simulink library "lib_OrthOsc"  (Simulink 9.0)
settings: Solver=ode45  StartTime=0.0  StopTime=10.0  RelTol=1e-3  EnableMultiTasking=on
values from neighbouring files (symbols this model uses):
  Tinit = 0.100    (= 0.1)    [TestOrthOscObjO_init.m]    (also in TestWaveMng_init.m)
  Tstep = 0.0005    [TestOrthOscObjO_init.m]    (also in TestWaveMng_init.m = 5e-05)
undefined symbols (not defined in the file or in its folder): Fmax, Fmin, Fnom, K, maxError, minMagn, src2genBus, Tg, TP, Tstep_
libraries: lib_T1Blocks_FB x5, lib_Conv x5, lib_Ortholator x2, lib_AngleVectorBlocks x2, lib_Inspc x1

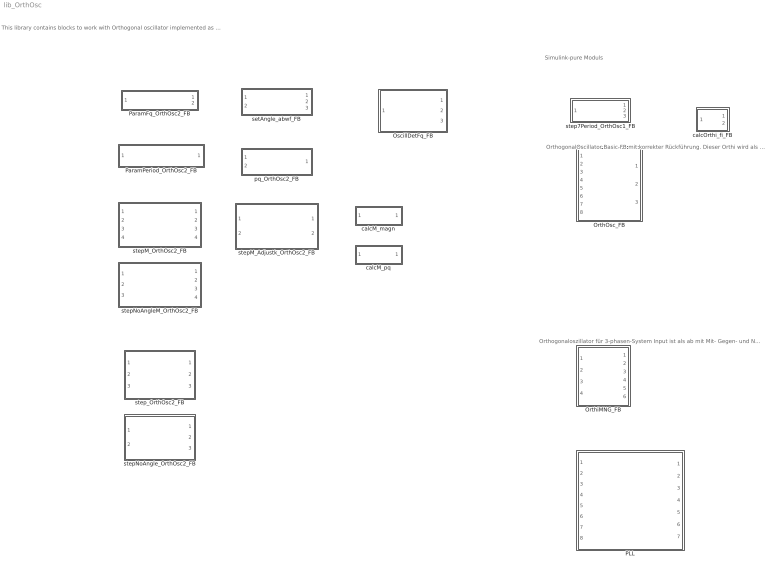
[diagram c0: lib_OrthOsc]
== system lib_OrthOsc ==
  note: Simulink-pure Moduls
  note: This library contains blocks to work with Orthogonal oscillator implemented as S-Function
  note: Orthogonaloszillator für 3-phasen-System Input ist als ab mit Mit- Gegen- und Nullsystem gegeben. Orthi separiert Gleichanteil (yG), Mitsystem(yM) und Gegensystem (yN) date=2016-03-04
  note: OrthogonalOscillator Basic-FB mit korrekter Rückführung. Dieser Orthi wird als Basis in den anderen FB verwendet.
  OrthOsc_FB : Subsystem
  OrthiMNG_FB : Subsystem
  OscillDetFq_FB : Subsystem
  PLL : Subsystem
  ParamFq_OrthOsc2_FB : Subsystem
  ParamPeriod_OrthOsc2_FB : Subsystem
  calcM_magn : Subsystem  TreatAsAtomicUnit=on
  calcM_pq : Subsystem  TreatAsAtomicUnit=on
  calcOrthi_fi_FB : Subsystem
  pq_OrthOsc2_FB : Subsystem
  setAngle_abwf_FB : Subsystem
  step7Period_OrthOsc1_FB : Subsystem
  stepM_Adjustk_OrthOsc2_FB : Subsystem  TreatAsAtomicUnit=on
  stepM_OrthOsc2_FB : Subsystem  TreatAsAtomicUnit=on
  stepNoAngleM_OrthOsc2_FB : Subsystem  TreatAsAtomicUnit=on
  stepNoAngle_OrthOsc2_FB : Subsystem
  step_OrthOsc2_FB : Subsystem  LoadFcn=src2genBus.lib_OrthOsc_genBus();

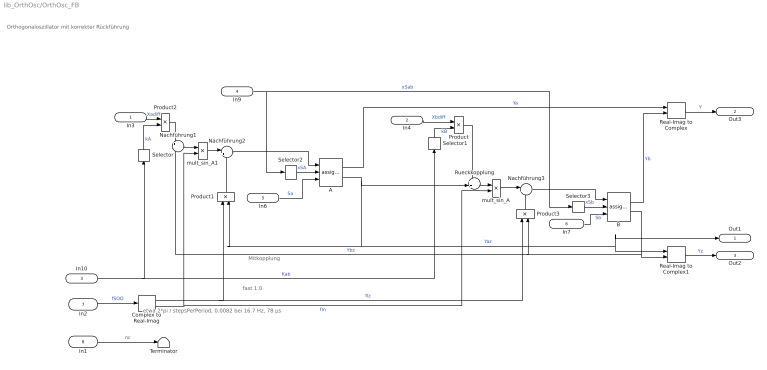
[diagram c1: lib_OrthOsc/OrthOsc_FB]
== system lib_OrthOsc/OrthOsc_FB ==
  note: Orthogonaloszillator mit korrekter Rückführung
  note: fast 1.0
  note: etwa 2*pi / stepsPerPeriod, 0.0082 bei 16.7 Hz, 78 µs
  note: Mitkopplung
  In3 : Inport
  In4 : Inport  Port=2
  In10 : Inport  Port=3  OutDataTypeStr=single  PortDimensions=2
  In9 : Inport  Port=4
  In6 : Inport  Port=5  OutDataTypeStr=boolean
  In7 : Inport  Port=6  OutDataTypeStr=boolean
  In2 : Inport  Port=7  OutDataTypeStr=single
  In1 : Inport  Port=8  OutDataTypeStr=boolean
  A : lib_T1Blocks_FB/assignS_OpC
  B : lib_T1Blocks_FB/assignS_OpC
  Complex to Real-Imag : ComplexToRealImag
  Nachführung1 : Sum  Inputs=+|-
  Nachführung2 : Sum  Inputs=|++
  Nachführung3 : Sum  Inputs=|++
  Product{,1..3} (4 alike) : Product
  Real-Imag to Complex : RealImagToComplex
  Real-Imag to Complex1 : RealImagToComplex
  Rueckkopplung : Sum  Inputs=++|
  Selector : Selector  InputPortWidth=2  IndexOptions=Index vector (dialog)  Indices=[1]  OutputSizes=1
  Selector1 : Selector  InputPortWidth=2  IndexOptions=Index vector (dialog)  Indices=[2]  OutputSizes=1
  Selector2 : Selector  InputPortWidth=2  IndexOptions=Index vector (dialog)  Indices=[1]  OutputSizes=1
  Selector3 : Selector  InputPortWidth=2  IndexOptions=Index vector (dialog)  Indices=[2]  OutputSizes=1
  Terminator : Terminator
  mult_sin_A : Product
  mult_sin_A1 : Product
  Out1 : Outport
  Out3 : Outport  Port=2
  Out2 : Outport  Port=3
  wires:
  In1/1 -> Terminator/1  "nc"
  In9/1 -> Selector2/1, Selector3/1  "xSab"
  In10/1 -> Selector1/1, Selector/1  "Kab"
  Real-Imag to Complex1/1 -> Out2/1  "Yz"
  B/1 -> Real-Imag to Complex/2  "Yb"
  Complex to Real-Imag/1 -> Product3/1, Product1/1  "fIz"
  Product3/1 -> Nachführung3/2
  Nachführung3/1 -> B/1
  Product1/1 -> Nachführung2/2
  Nachführung2/1 -> A/1
  Selector2/1 -> A/2  "xSA"
  Selector3/1 -> B/2  "xSb"
  In7/1 -> B/3  "Sb"
  Selector1/1 -> Product/2  "kB"
  In4/1 -> Product/1  "Xbdiff"
  In6/1 -> A/3  "Sa"
  Selector/1 -> Product2/2  "kA"
  B/2 -> Real-Imag to Complex1/2, Product3/2, Nachführung1/2  "Ybz"
  A/1 -> Real-Imag to Complex/1  "Ya"
  mult_sin_A/1 -> Nachführung3/1
  Rueckkopplung/1 -> mult_sin_A/1
  In2/1 -> Complex to Real-Imag/1  "fSOO"
  Product/1 -> Rueckkopplung/1
  In3/1 -> Product2/1  "Xadiff"
  Product2/1 -> Nachführung1/1
  A/2 -> Rueckkopplung/2, Real-Imag to Complex1/1, Out1/1, Product1/2  "Yaz"
  Nachführung1/1 -> mult_sin_A1/1
  mult_sin_A1/1 -> Nachführung2/1
  Real-Imag to Complex/1 -> Out3/1  "Y"
  Complex to Real-Imag/2 -> mult_sin_A/2, mult_sin_A1/2  "fIn"

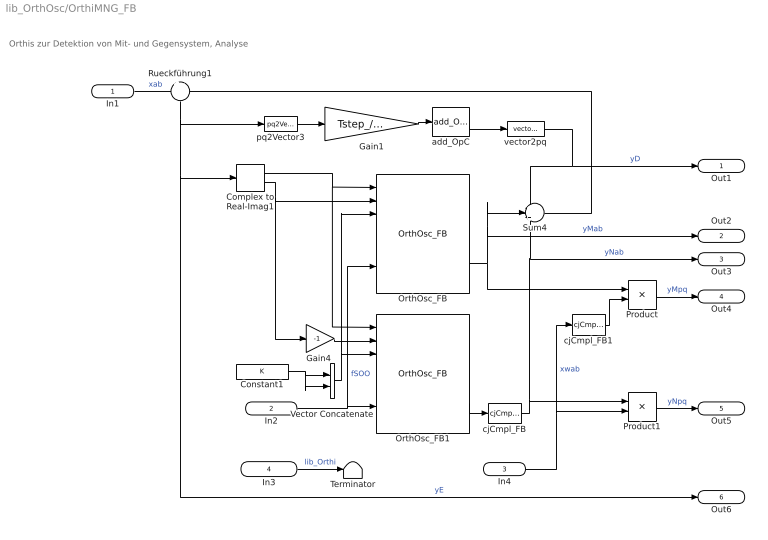
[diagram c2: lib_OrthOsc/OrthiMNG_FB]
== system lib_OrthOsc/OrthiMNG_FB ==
  note: Orthis zur Detektion von Mit- und Gegensystem, Analyse
  In1 : Inport  OutDataTypeStr=single
  In2 : Inport  Port=2  OutDataTypeStr=single
  In4 : Inport  Port=3  OutDataTypeStr=single
  In3 : Inport  Port=4  OutDataTypeStr=boolean
  Complex to Real-Imag1 : ComplexToRealImag
  Constant1 : Constant  Value=K  OutDataTypeStr=single
  Gain1 : Gain  Gain=Tstep_/Tg
  Gain4 : Gain  Gain=-1
  OrthOsc_FB : lib_Ortholator/OrthOsc_FB
  OrthOsc_FB1 : lib_Ortholator/OrthOsc_FB
  Product : Product
  Product1 : Product
  Rueckführung1 : Sum  Inputs=+-
  Sum4 : Sum  Inputs=+++
  Terminator : Terminator
  Vector Concatenate : Concatenate
  add_OpC : lib_T1Blocks_FB/add_OpC  y0=0
  cjCmpl_FB : lib_Conv/cjCmpl_FB
  cjCmpl_FB1 : lib_Conv/cjCmpl_FB
  pq2Vector3 : lib_Conv/pq2Vector  SystemSampleTime=-1
  vector2pq : lib_Conv/vector2pq  SystemSampleTime=-1
  Out1 : Outport  OutDataTypeStr=single
  Out2 : Outport  Port=2  OutDataTypeStr=single
  Out3 : Outport  Port=3  OutDataTypeStr=single
  Out4 : Outport  Port=4  OutDataTypeStr=single
  Out5 : Outport  Port=5  OutDataTypeStr=single
  Out6 : Outport  Port=6  OutDataTypeStr=single
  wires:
  Product1/1 -> Out5/1  "yNpq"
  Product/1 -> Out4/1  "yMpq"
  In4/1 -> Product1/2, cjCmpl_FB1/1  "xwab"
  cjCmpl_FB1/1 -> Product/2
  OrthOsc_FB1/3 -> cjCmpl_FB/1
  cjCmpl_FB/1 -> Product1/1, Sum4/3, Out3/1  "yNab"
  Sum4/1 -> Rueckführung1/2
  OrthOsc_FB/3 -> Product/1, Out2/1, Sum4/2  "yMab"
  In2/1 -> OrthOsc_FB/7, OrthOsc_FB1/7  "fSOO"
  Gain1/1 -> add_OpC/1
  In1/1 -> Rueckführung1/1  "xab"
  Rueckführung1/1 -> Out6/1, Complex to Real-Imag1/1, pq2Vector3/1  "yE"
  Vector Concatenate/1 -> OrthOsc_FB1/3, OrthOsc_FB/3
  vector2pq/1 -> Out1/1, Sum4/1  "yD"
  Complex to Real-Imag1/1 -> OrthOsc_FB1/1, OrthOsc_FB/1
  pq2Vector3/1 -> Gain1/1
  add_OpC/2 -> vector2pq/1
  Complex to Real-Imag1/2 -> Gain4/1, OrthOsc_FB/2
  Gain4/1 -> OrthOsc_FB1/2
  Constant1/1 -> Vector Concatenate/2, Vector Concatenate/1
  In3/1 -> Terminator/1  "lib_Orthi"

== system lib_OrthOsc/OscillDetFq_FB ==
  In1 : Inport  OutDataTypeStr=single  PortDimensions=1
  SFunc : S-Function  LoadFcn=src2genBus.lib_OrthOsc_genBus();  FunctionName=step_OscillDetFq_FB_SfH  Parameters=ident Tstep dxstart dxmin amplMin stepNom stepMax  SFunctionDeploymentMode=off  EnableBusSupport=off
  Out4 : Outport  OutDataTypeStr=uint32  SampleTime=Tinit
  Out1 : Outport  Port=2  OutDataTypeStr=uint32
  Out3 : Outport  Port=3  OutDataTypeStr=single
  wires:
  SFunc/2 -> Out1/1  "thiz"
  In1/1 -> SFunc/1  "X"
  SFunc/3 -> Out3/1  "nSteps"
  SFunc/1 -> Out4/1  "OscillDetFq_FB"

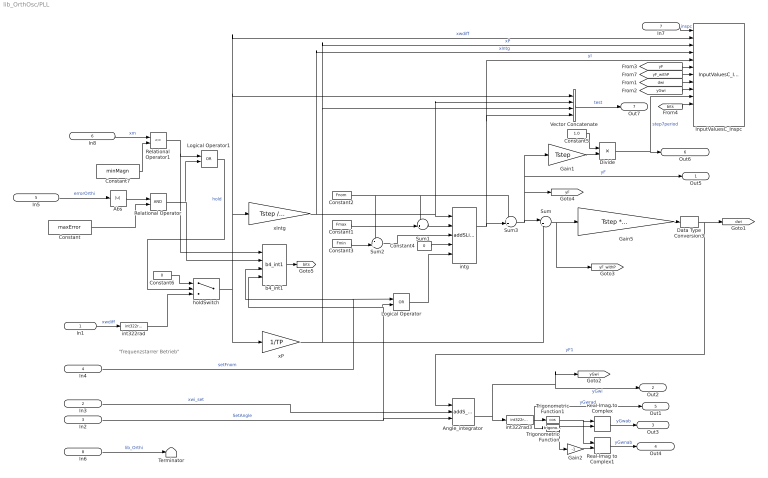
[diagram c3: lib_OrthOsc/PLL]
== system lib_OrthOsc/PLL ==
  note: "frequenzstarrer Betrieb"
  In1 : Inport
  In3 : Inport  Port=2  OutDataTypeStr=int32
  In2 : Inport  Port=3  OutDataTypeStr=boolean
  In4 : Inport  Port=4  OutDataTypeStr=boolean
  In5 : Inport  Port=5  OutDataTypeStr=single  PortDimensions=1
  In8 : Inport  Port=6  OutDataTypeStr=single  PortDimensions=1
  In7 : Inport  Port=7  OutDataTypeStr=P_FBaccess_Inspc  PortDimensions=1  SampleTime=Tstep
  In6 : Inport  Port=8  OutDataTypeStr=boolean
  Abs : Abs
  Angle_integrator : lib_T1Blocks_FB/addS_OpC
  Constant : Constant  Value=maxError
  Constant1 : Constant  Value=Fmax  OutDataTypeStr=single
  Constant2 : Constant  Value=Fnom  OutDataTypeStr=single
  Constant3 : Constant  Value=Fmin  OutDataTypeStr=single
  Constant4 : Constant  Value=0  OutDataTypeStr=single
  Constant5 : Constant  Value=1.0  OutDataTypeStr=single
  Constant6 : Constant  Value=0  OutDataTypeStr=single
  Constant7 : Constant  Value=minMagn
  Data Type Conversion3 : DataTypeConversion  OutDataTypeStr=int32
  Divide : Product  Inputs=*/
  Gain1 : Gain  Gain=Tstep
  Gain2 : Gain  Gain=-1
  Gain5 : Gain  Gain=Tstep * 65536 * 65536
  InputValuesC_Inspc : lib_Inspc/InputValuesC_Inspc  nameRefl=nameInspc  n1='wxdiff_rad'  n2='xP'  n3='xIntg'  n4='yIntg'  n5='yF'  n6='yF_withP'  n7='dwi'  n8='yGwi'  n9='step7period'  n10='hold_setG_setF_err_magn'  n11=''  n12=''
  Logical Operator : Logic  Operator=OR  IconShape=distinctive  AllPortsSameDT=off  OutDataTypeStr=boolean
  Logical Operator1 : Logic  Operator=OR  AllPortsSameDT=off  OutDataTypeStr=boolean
  Real-Imag to Complex : RealImagToComplex
  Real-Imag to Complex1 : RealImagToComplex
  Relational Operator : RelationalOperator  OutDataTypeStr=boolean
  Relational Operator1 : RelationalOperator  Operator=<=  OutDataTypeStr=boolean
  Sum : Sum  Inputs=|++
  Sum1 : Sum  Inputs=-+|
  Sum2 : Sum  Inputs=-+|
  Sum3 : Sum  Inputs=++|
  Terminator : Terminator
  Trigonometric Function : Trigonometry
  Trigonometric Function1 : Trigonometry  Operator=cos
  Vector Concatenate : Concatenate  NumInputs=4
  b4_int1 : lib_Conv/b4_int1  b0bit=0  b1bit=1  b2bit=2  b3bit=3
  holdSwitch : Switch
  int322rad : lib_AngleVectorBlocks/int322rad
  int322rad3 : lib_AngleVectorBlocks/int322rad
  intg : lib_T1Blocks_FB/addSLim_OpC
  xIntg : Gain  Gain=Tstep / Tintg
  xP : Gain  Gain=1/TP
  Out5 : Outport  OutDataTypeStr=single  PortDimensions=1
  Out2 : Outport  Port=2  OutDataTypeStr=int32  PortDimensions=1
  Out3 : Outport  Port=3  OutDataTypeStr=single  PortDimensions=1
  Out4 : Outport  Port=4  OutDataTypeStr=single  PortDimensions=1
  Out1 : Outport  Port=5  OutDataTypeStr=single  PortDimensions=1
  Out6 : Outport  Port=6  OutDataTypeStr=single  PortDimensions=1
  Out7 : Outport  Port=7  OutDataTypeStr=single  PortDimensions=4
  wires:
  [bits] -> InputValuesC_Inspc/11
  b4_int1/1 -> [bits]
  [yF] -> InputValuesC_Inspc/6
  In8/1 -> Relational Operator1/1  "xm"
  Relational Operator/1 -> b4_int1/2, Logical Operator1/2
  Relational Operator1/1 -> b4_int1/1, Logical Operator1/1
  Constant7/1 -> Relational Operator1/2
  Constant/1 -> Relational Operator/2
  Abs/1 -> Relational Operator/1
  In5/1 -> Abs/1  "errorOrthi"
  [yGwi] -> InputValuesC_Inspc/9
  [dwi] -> InputValuesC_Inspc/8
  [yF_withP] -> InputValuesC_Inspc/7
  In7/1 -> InputValuesC_Inspc/1  "inspc"
  int322rad/1 -> holdSwitch/3
  Constant6/1 -> holdSwitch/1
  Vector Concatenate/1 -> Out7/1  "test"
  In6/1 -> Terminator/1  "lib_Orthi"
  holdSwitch/1 -> Vector Concatenate/1, InputValuesC_Inspc/2, xIntg/1, xP/1  "xwdiff"
  Logical Operator1/1 -> holdSwitch/2  "hold"
  In4/1 -> Logical Operator/1, b4_int1/3  "setFnom"
  Logical Operator/1 -> intg/5
  Divide/1 -> Out6/1, InputValuesC_Inspc/10  "step7period"
  Constant5/1 -> Divide/1
  Gain1/1 -> Divide/2
  In3/1 -> Angle_integrator/2  "xwi_set"
  In2/1 -> b4_int1/4, Logical Operator/2, Angle_integrator/3  "SetAngle"
  xIntg/1 -> Vector Concatenate/2, intg/1, InputValuesC_Inspc/4  "xIntg"
  xP/1 -> Sum/2, Vector Concatenate/3, InputValuesC_Inspc/3  "xP"
  In1/1 -> int322rad/1  "xwdiff"
  Constant4/1 -> intg/4
  Constant3/1 -> Sum2/2
  Sum2/1 -> intg/3
  Sum1/1 -> intg/2
  Constant2/1 -> Sum3/1, Sum1/1, Sum2/1
  Sum/1 -> Gain5/1, [yF_withP]
  Data Type Conversion3/1 -> Angle_integrator/1, [dwi]  "yF1"
  Constant1/1 -> Sum1/2
  intg/1 -> Sum3/2, Vector Concatenate/4, InputValuesC_Inspc/5  "yI"
  Gain5/1 -> Data Type Conversion3/1
  Real-Imag to Complex1/1 -> Out4/1  "yGwnab"
  Real-Imag to Complex/1 -> Out3/1  "yGwab"
  Gain2/1 -> Real-Imag to Complex1/2
  Trigonometric Function/1 -> Real-Imag to Complex/2, Gain2/1
  Trigonometric Function1/1 -> Real-Imag to Complex/1, Real-Imag to Complex1/1
  int322rad3/1 -> Trigonometric Function1/1, Trigonometric Function/1, Out1/1  "yGwrad"
  Angle_integrator/2 -> int322rad3/1, Out2/1, [yGwi]  "yGwi"
  Sum3/1 -> Out5/1, Gain1/1, [yF], Sum/1  "yF"

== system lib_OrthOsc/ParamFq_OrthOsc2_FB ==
  In1 : Inport  OutDataTypeStr=single
  param1_myOrthOsc : S-Function  FunctionName=setFq_Param_OrthOsc2_FB_SfH  Parameters=identObj Tstep TstepOrth m_nom  SFunctionDeploymentMode=off  EnableBusSupport=off
  Out2 : Outport  OutDataTypeStr=uint32  SampleTime=Tinit
  Out1 : Outport  Port=2  OutDataTypeStr=uint32  SampleTime=Tstep
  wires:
  In1/1 -> param1_myOrthOsc/1  "fq"
  param1_myOrthOsc/1 -> Out2/1  "Param_OrthOsc2_FB"
  param1_myOrthOsc/2 -> Out1/1  "thiz"

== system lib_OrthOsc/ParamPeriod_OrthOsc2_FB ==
  In1 : Inport  OutDataTypeStr=single
  sfn : S-Function  FunctionName=setPeriod_Param_OrthOsc2_FB_SfH  Parameters=identObj Tstep TstepOrth m_nom  SFunctionDeploymentMode=off  EnableBusSupport=off
  Out2 : Outport  OutDataTypeStr=uint32
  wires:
  sfn/1 -> Out2/1  "Param_OrthOsc2_FB"
  In1/1 -> sfn/1  "nPeriod"

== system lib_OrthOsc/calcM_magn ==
  In1 : Inport  OutDataTypeStr=uint32  Partition=on  PartitionDimension=1  PartitionWidth=1  PartitionOffset=0
  For Each : ForEach  DisableCoverage=on  IndexMode=One-based
  calcMagn_Orthi2_FB : S-Function  FunctionName=calcMagn_OrthOsc2_FB_SfH  SFunctionDeploymentMode=off  EnableBusSupport=off
  Out3 : Outport  OutDataTypeStr=single  ConcatenationDimension=1
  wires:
  In1/1 -> calcMagn_Orthi2_FB/1  "thiz"
  calcMagn_Orthi2_FB/1 -> Out3/1  "ym"

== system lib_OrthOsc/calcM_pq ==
  In1 : Inport  OutDataTypeStr=uint32  Partition=on  PartitionDimension=1  PartitionWidth=1  PartitionOffset=0
  For Each : ForEach  DisableCoverage=on  IndexMode=One-based
  step_Orthi2_FB : S-Function  FunctionName=calcpq_OrthOsc2_FB_SfH  SFunctionDeploymentMode=off  EnableBusSupport=off
  Out3 : Outport  OutDataTypeStr=single  ConcatenationDimension=1
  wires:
  In1/1 -> step_Orthi2_FB/1  "thiz"
  step_Orthi2_FB/1 -> Out3/1  "ypq"

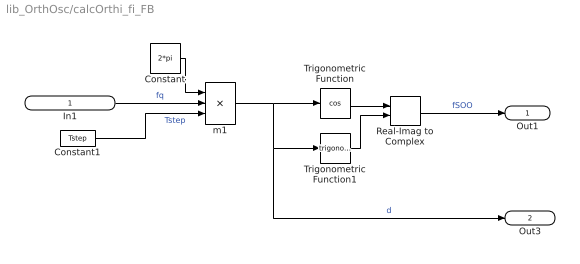
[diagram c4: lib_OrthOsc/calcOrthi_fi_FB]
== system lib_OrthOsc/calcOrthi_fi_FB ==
  In1 : Inport  OutDataTypeStr=single
  Constant : Constant  Value=2*pi  OutDataTypeStr=single
  Constant1 : Constant  Value=Tstep  OutDataTypeStr=single
  Real-Imag to Complex : RealImagToComplex
  Trigonometric Function : Trigonometry  Operator=cos
  Trigonometric Function1 : Trigonometry
  m1 : Product  Inputs=***
  Out1 : Outport
  Out3 : Outport  Port=2
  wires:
  Constant1/1 -> m1/3  "Tstep"
  Constant/1 -> m1/1
  m1/1 -> Trigonometric Function/1, Trigonometric Function1/1, Out3/1  "d"
  In1/1 -> m1/2  "fq"
  Real-Imag to Complex/1 -> Out1/1  "fSOO"
  Trigonometric Function1/1 -> Real-Imag to Complex/2
  Trigonometric Function/1 -> Real-Imag to Complex/1

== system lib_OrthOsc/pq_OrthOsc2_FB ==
  In3 : Inport  OutDataTypeStr=uint32
  In2 : Inport  Port=2  OutDataTypeStr=single
  calcpq_OrthOsc2_FB : S-Function  FunctionName=calcpq_OrthOsc2_FB_SfH  SFunctionDeploymentMode=off  EnableBusSupport=off
  thiz_Angle_abwmf_FB : Outport  OutDataTypeStr=single
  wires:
  In3/1 -> calcpq_OrthOsc2_FB/1  "thiz_OrthOs2_FB"
  In2/1 -> calcpq_OrthOsc2_FB/2  "step"
  calcpq_OrthOsc2_FB/1 -> thiz_Angle_abwmf_FB/1  "pq"

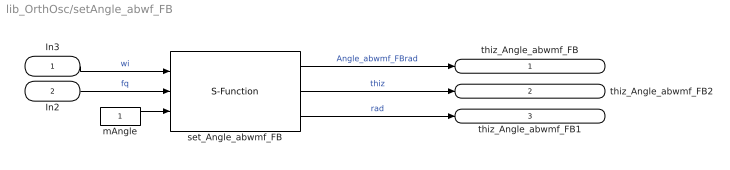
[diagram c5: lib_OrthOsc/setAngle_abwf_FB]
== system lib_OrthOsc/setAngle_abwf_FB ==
  In3 : Inport  OutDataTypeStr=int32
  In2 : Inport  Port=2  OutDataTypeStr=single
  mAngle : Constant  OutDataTypeStr=single
  set_Angle_abwmf_FB : S-Function  FunctionName=set_Angle_abwmf_FB_SfH  Parameters=identObj  SFunctionDeploymentMode=off  EnableBusSupport=off
  thiz_Angle_abwmf_FB : Outport  OutDataTypeStr=uint32  SampleTime=Tinit
  thiz_Angle_abwmf_FB2 : Outport  Port=2  OutDataTypeStr=uint32  SampleTime=Tstep
  thiz_Angle_abwmf_FB1 : Outport  Port=3  OutDataTypeStr=single
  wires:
  In3/1 -> set_Angle_abwmf_FB/1  "wi"
  In2/1 -> set_Angle_abwmf_FB/2  "fq"
  mAngle/1 -> set_Angle_abwmf_FB/3
  set_Angle_abwmf_FB/1 -> thiz_Angle_abwmf_FB/1  "Angle_abwmf_FBrad"
  set_Angle_abwmf_FB/3 -> thiz_Angle_abwmf_FB1/1  "rad"
  set_Angle_abwmf_FB/2 -> thiz_Angle_abwmf_FB2/1  "thiz"

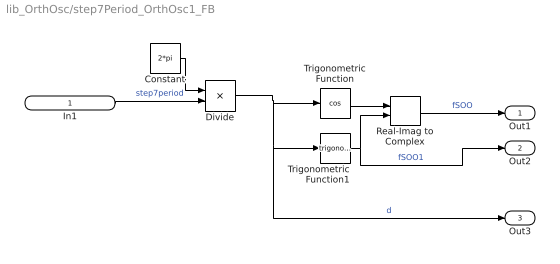
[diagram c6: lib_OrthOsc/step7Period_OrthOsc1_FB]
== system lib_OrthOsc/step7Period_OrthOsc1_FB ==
  In1 : Inport  OutDataTypeStr=single
  Constant : Constant  Value=2*pi  OutDataTypeStr=single
  Divide : Product  Inputs=*/
  Real-Imag to Complex : RealImagToComplex
  Trigonometric Function : Trigonometry  Operator=cos
  Trigonometric Function1 : Trigonometry
  Out1 : Outport
  Out2 : Outport  Port=2
  Out3 : Outport  Port=3
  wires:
  Trigonometric Function/1 -> Real-Imag to Complex/1
  Trigonometric Function1/1 -> Real-Imag to Complex/2, Out2/1  "fSOO1"
  Real-Imag to Complex/1 -> Out1/1  "fSOO"
  In1/1 -> Divide/2  "step7period"
  Divide/1 -> Out3/1, Trigonometric Function1/1, Trigonometric Function/1  "d"
  Constant/1 -> Divide/1

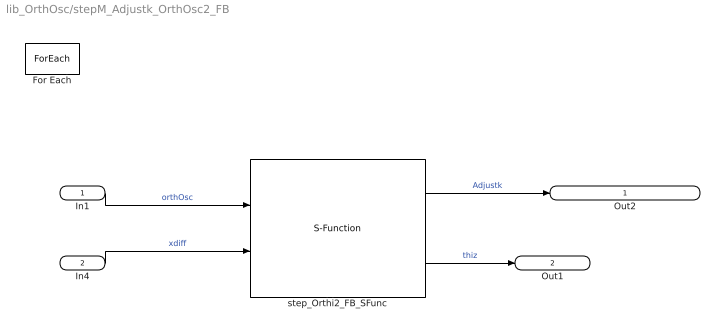
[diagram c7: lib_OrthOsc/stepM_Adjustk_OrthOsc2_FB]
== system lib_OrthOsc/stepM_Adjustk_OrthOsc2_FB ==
  In1 : Inport  OutDataTypeStr=uint32  PortDimensions=1  Partition=on  PartitionDimension=1  PartitionWidth=1  PartitionOffset=0
  In4 : Inport  Port=2  OutDataTypeStr=single  Partition=on  PartitionDimension=1  PartitionWidth=1  PartitionOffset=0
  For Each : ForEach  DisableCoverage=on  IndexMode=One-based
  step_Orthi2_FB_SFunc : S-Function  LoadFcn=src2genBus.lib_OrthOsc_genBus();  FunctionName=step_Adjustk_OrthOsc2_FB_SfH  Parameters=ident max_e kHi kNormal Tstep Tdecay  SFunctionDeploymentMode=off  EnableBusSupport=off
  Out2 : Outport  OutDataTypeStr=uint32  ConcatenationDimension=1
  Out1 : Outport  Port=2  OutDataTypeStr=uint32  ConcatenationDimension=1
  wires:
  In4/1 -> step_Orthi2_FB_SFunc/2  "xdiff"
  In1/1 -> step_Orthi2_FB_SFunc/1  "orthOsc"
  step_Orthi2_FB_SFunc/2 -> Out1/1  "thiz"
  step_Orthi2_FB_SFunc/1 -> Out2/1  "Adjustk"

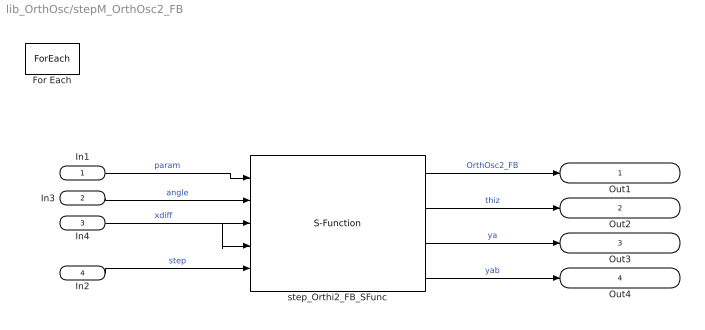
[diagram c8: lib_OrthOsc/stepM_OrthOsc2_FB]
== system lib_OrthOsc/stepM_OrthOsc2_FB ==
  In1 : Inport  OutDataTypeStr=uint32  PortDimensions=1
  In3 : Inport  Port=2  OutDataTypeStr=uint32
  In4 : Inport  Port=3  OutDataTypeStr=single  Partition=on  PartitionDimension=1  PartitionWidth=1  PartitionOffset=0
  In2 : Inport  Port=4  OutDataTypeStr=uint32  PortDimensions=1
  For Each : ForEach  DisableCoverage=on  IndexMode=One-based
  step_Orthi2_FB_SFunc : S-Function  LoadFcn=src2genBus.lib_OrthOsc_genBus();  FunctionName=step_OrthOsc2_FB_SfH  Parameters=ident kA kB  SFunctionDeploymentMode=off  EnableBusSupport=off
  Out1 : Outport  OutDataTypeStr=uint32  SampleTime=Tinit  ConcatenationDimension=1
  Out2 : Outport  Port=2  OutDataTypeStr=uint32  SampleTime=Tstep  ConcatenationDimension=1
  Out3 : Outport  Port=3  OutDataTypeStr=single  ConcatenationDimension=1
  Out4 : Outport  Port=4  OutDataTypeStr=single  ConcatenationDimension=1
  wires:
  In3/1 -> step_Orthi2_FB_SFunc/2  "angle"
  In1/1 -> step_Orthi2_FB_SFunc/1  "param"
  step_Orthi2_FB_SFunc/1 -> Out1/1  "OrthOsc2_FB"
  In4/1 -> step_Orthi2_FB_SFunc/4, step_Orthi2_FB_SFunc/3  "xdiff"
  step_Orthi2_FB_SFunc/3 -> Out3/1  "ya"
  step_Orthi2_FB_SFunc/4 -> Out4/1  "yab"
  step_Orthi2_FB_SFunc/2 -> Out2/1  "thiz"
  In2/1 -> step_Orthi2_FB_SFunc/5  "step"

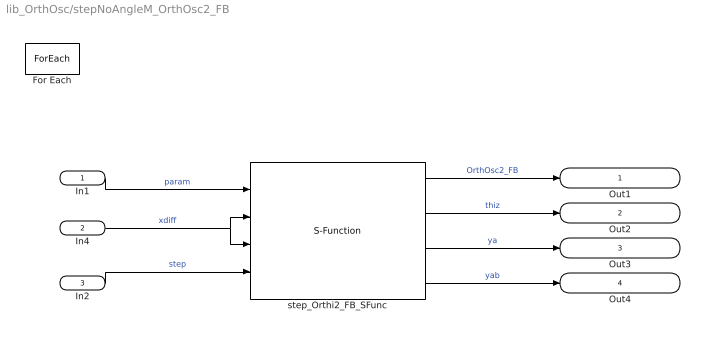
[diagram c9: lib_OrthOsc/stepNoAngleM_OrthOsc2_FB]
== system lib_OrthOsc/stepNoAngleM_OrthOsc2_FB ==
  In1 : Inport  OutDataTypeStr=uint32  PortDimensions=1
  In4 : Inport  Port=2  OutDataTypeStr=single  Partition=on  PartitionDimension=1  PartitionWidth=1  PartitionOffset=0
  In2 : Inport  Port=3  OutDataTypeStr=uint32  PortDimensions=1
  For Each : ForEach  DisableCoverage=on  IterateSubsysMaskParameter=off,off,off  IndexMode=One-based
  step_Orthi2_FB_SFunc : S-Function  LoadFcn=src2genBus.lib_OrthOsc_genBus();  FunctionName=stepNoAngle_OrthOsc2_FB_SfH  Parameters=ident kA kB  SFunctionDeploymentMode=off  EnableBusSupport=off
  Out1 : Outport  OutDataTypeStr=uint32  SampleTime=Tinit  ConcatenationDimension=1
  Out2 : Outport  Port=2  OutDataTypeStr=uint32  SampleTime=Tstep  ConcatenationDimension=1
  Out3 : Outport  Port=3  OutDataTypeStr=single  ConcatenationDimension=1
  Out4 : Outport  Port=4  OutDataTypeStr=single  ConcatenationDimension=1
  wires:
  step_Orthi2_FB_SFunc/4 -> Out4/1  "yab"
  step_Orthi2_FB_SFunc/3 -> Out3/1  "ya"
  In4/1 -> step_Orthi2_FB_SFunc/3, step_Orthi2_FB_SFunc/2  "xdiff"
  step_Orthi2_FB_SFunc/1 -> Out1/1  "OrthOsc2_FB"
  In1/1 -> step_Orthi2_FB_SFunc/1  "param"
  step_Orthi2_FB_SFunc/2 -> Out2/1  "thiz"
  In2/1 -> step_Orthi2_FB_SFunc/4  "step"

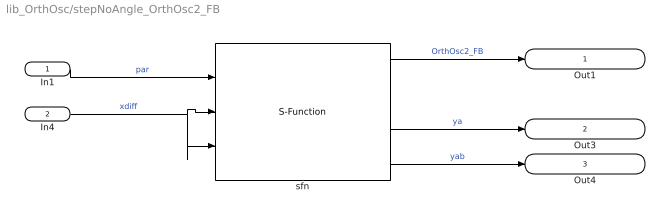
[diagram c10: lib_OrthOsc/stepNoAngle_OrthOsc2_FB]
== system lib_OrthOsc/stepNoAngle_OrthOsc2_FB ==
  In1 : Inport  OutDataTypeStr=uint32  PortDimensions=1
  In4 : Inport  Port=2  OutDataTypeStr=single
  sfn : S-Function  LoadFcn=src2genBus.lib_OrthOsc_genBus();  FunctionName=stepNoAngle_OrthOsc2_FB_SfH  Parameters=ident kA kB  SFunctionDeploymentMode=off  EnableBusSupport=off
  Out1 : Outport  OutDataTypeStr=uint32
  Out3 : Outport  Port=2  OutDataTypeStr=single
  Out4 : Outport  Port=3  OutDataTypeStr=single
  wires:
  In1/1 -> sfn/1  "par"
  sfn/1 -> Out1/1  "OrthOsc2_FB"
  In4/1 -> sfn/2, sfn/3  "xdiff"
  sfn/3 -> Out3/1  "ya"
  sfn/4 -> Out4/1  "yab"

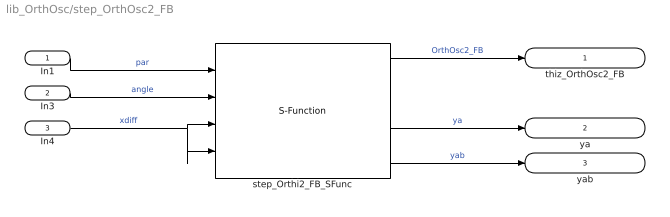
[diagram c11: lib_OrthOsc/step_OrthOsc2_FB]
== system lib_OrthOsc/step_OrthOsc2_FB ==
  In1 : Inport  OutDataTypeStr=uint32  PortDimensions=1
  In3 : Inport  Port=2  OutDataTypeStr=uint32
  In4 : Inport  Port=3  OutDataTypeStr=single
  step_Orthi2_FB_SFunc : S-Function  LoadFcn=src2genBus.lib_OrthOsc_genBus();  FunctionName=step_OrthOsc2_FB_SfH  Parameters=ident kA kB  SFunctionDeploymentMode=off  EnableBusSupport=off
  thiz_OrthOsc2_FB : Outport  OutDataTypeStr=uint32
  ya : Outport  Port=2  OutDataTypeStr=single
  yab : Outport  Port=3  OutDataTypeStr=single
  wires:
  step_Orthi2_FB_SFunc/4 -> yab/1  "yab"
  step_Orthi2_FB_SFunc/3 -> ya/1  "ya"
  In4/1 -> step_Orthi2_FB_SFunc/4, step_Orthi2_FB_SFunc/3  "xdiff"
  step_Orthi2_FB_SFunc/1 -> thiz_OrthOsc2_FB/1  "OrthOsc2_FB"
  In1/1 -> step_Orthi2_FB_SFunc/1  "par"
  In3/1 -> step_Orthi2_FB_SFunc/2  "angle"
